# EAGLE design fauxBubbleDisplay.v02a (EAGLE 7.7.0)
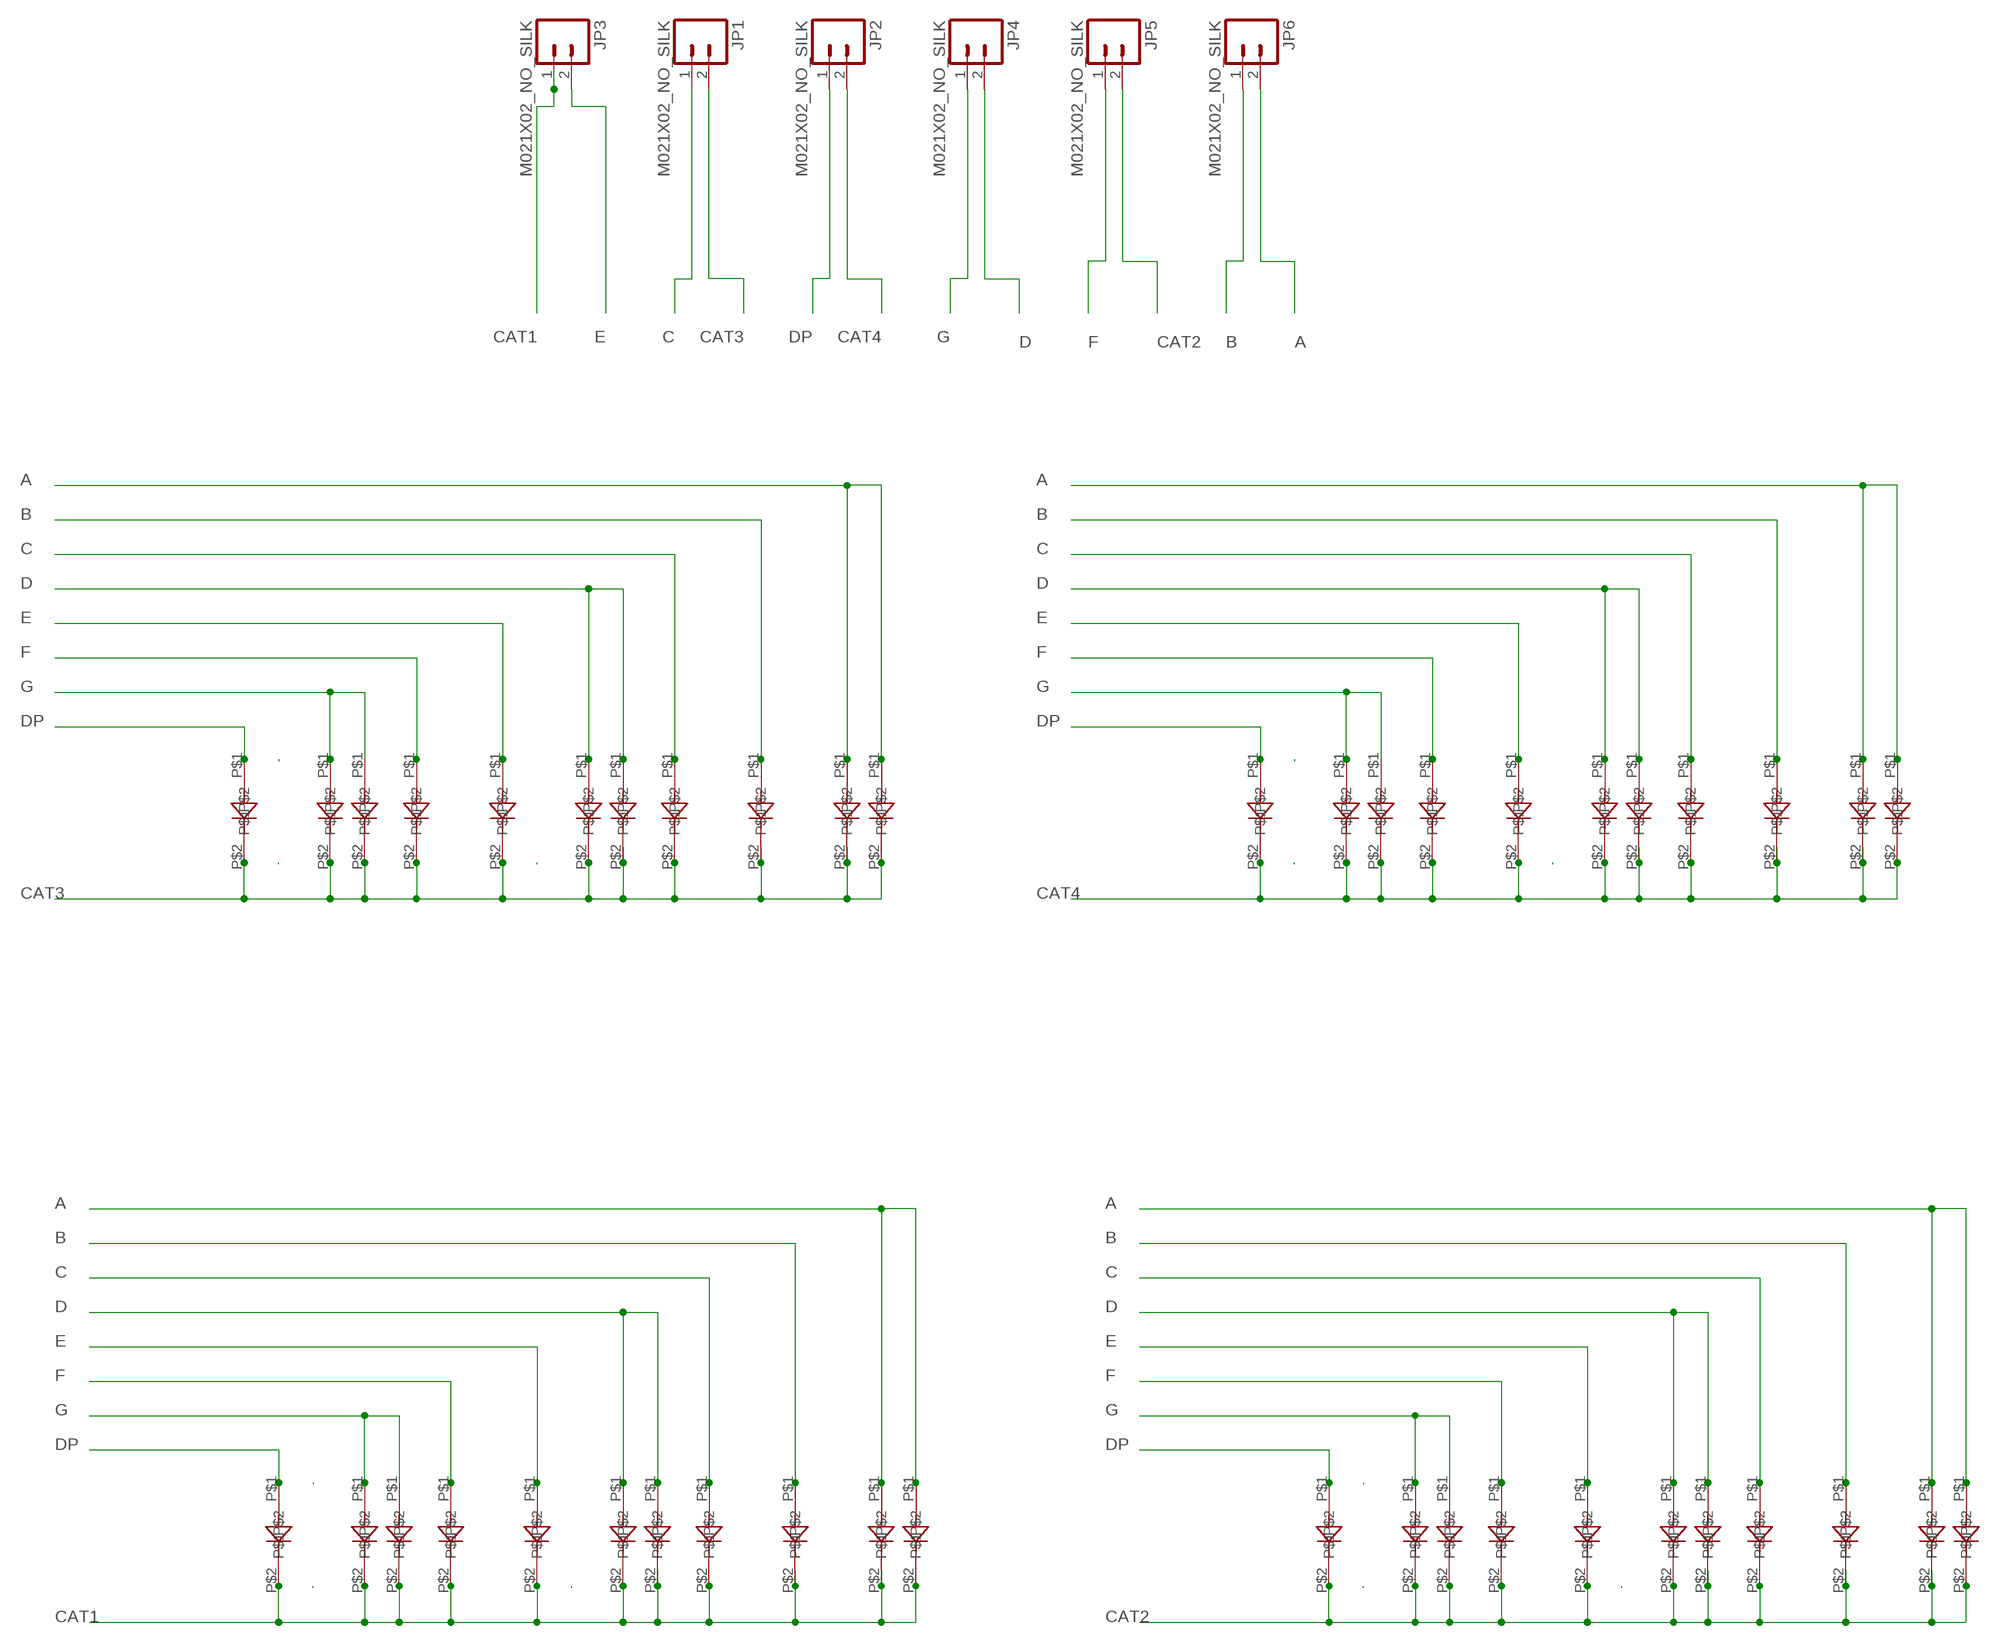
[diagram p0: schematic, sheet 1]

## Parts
JP1  M021X02_NO_SILK  [1X02_NO_SILK]
JP2  M021X02_NO_SILK  [1X02_NO_SILK]
JP3  M021X02_NO_SILK  [1X02_NO_SILK]
JP4  M021X02_NO_SILK  [1X02_NO_SILK]
JP5  M021X02_NO_SILK  [1X02_NO_SILK]
JP6  M021X02_NO_SILK  [1X02_NO_SILK]
U$1  LX201  [LX201]
U$2  LX201  [LX201]
U$3  LX201  [LX201]
U$4  LX201  [LX201]
U$5  LX201  [LX201]
U$6  LX201  [LX201]
U$7  LX201  [LX201]
U$8  LX201  [LX201]
U$9  LX201  [LX201]
U$10  LX201  [LX201]
U$11  LX201  [LX201]
U$12  LX201  [LX201]
U$13  LX201  [LX201]
U$14  LX201  [LX201]
U$15  LX201  [LX201]
U$16  LX201  [LX201]
U$17  LX201  [LX201]
U$18  LX201  [LX201]
U$19  LX201  [LX201]
U$20  LX201  [LX201]
U$21  LX201  [LX201]
U$22  LX201  [LX201]
U$23  LX201  [LX201]
U$24  LX201  [LX201]
U$25  LX201  [LX201]
U$26  LX201  [LX201]
U$27  LX201  [LX201]
U$28  LX201  [LX201]
U$29  LX201  [LX201]
U$30  LX201  [LX201]
U$31  LX201  [LX201]
U$32  LX201  [LX201]
U$33  LX201  [LX201]
U$34  LX201  [LX201]
U$35  LX201  [LX201]
U$36  LX201  [LX201]
U$37  LX201  [LX201]
U$38  LX201  [LX201]
U$39  LX201  [LX201]
U$40  LX201  [LX201]
U$41  LX201  [LX201]
U$42  LX201  [LX201]
U$43  LX201  [LX201]
U$44  LX201  [LX201]

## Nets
A: JP6.2 U$15.P$1 U$16.P$1 U$21.P$1 U$22.P$1 U$32.P$1 U$33.P$1 U$43.P$1 U$44.P$1
B: JP6.1 U$13.P$1 U$20.P$1 U$31.P$1 U$42.P$1
C: JP1.1 U$11.P$1 U$19.P$1 U$30.P$1 U$41.P$1
CAT1: JP3.1 U$1.P$2 U$2.P$2 U$4.P$2 U$5.P$2 U$7.P$2 U$9.P$2 U$10.P$2 U$11.P$2 U$13.P$2 U$15.P$2 U$16.P$2
CAT2: JP5.2 U$23.P$2 U$24.P$2 U$25.P$2 U$26.P$2 U$27.P$2 U$28.P$2 U$29.P$2 U$30.P$2 U$31.P$2 U$32.P$2 U$33.P$2
CAT3: JP1.2 U$3.P$2 U$6.P$2 U$8.P$2 U$12.P$2 U$14.P$2 U$17.P$2 U$18.P$2 U$19.P$2 U$20.P$2 U$21.P$2 U$22.P$2
CAT4: JP2.2 U$34.P$2 U$35.P$2 U$36.P$2 U$37.P$2 U$38.P$2 U$39.P$2 U$40.P$2 U$41.P$2 U$42.P$2 U$43.P$2 U$44.P$2
D: JP4.2 U$9.P$1 U$10.P$1 U$17.P$1 U$18.P$1 U$28.P$1 U$29.P$1 U$39.P$1 U$40.P$1
DP: JP2.1 U$4.P$1 U$8.P$1 U$25.P$1 U$36.P$1
E: JP3.2 U$7.P$1 U$14.P$1 U$27.P$1 U$38.P$1
F: JP5.1 U$5.P$1 U$12.P$1 U$26.P$1 U$37.P$1
G: JP4.1 U$1.P$1 U$2.P$1 U$3.P$1 U$6.P$1 U$23.P$1 U$24.P$1 U$34.P$1 U$35.P$1

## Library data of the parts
JP1-JP6 = SparkFun-Connectors:M02: Standard 2-pin 0.1" header. Use with
U$1-U$44 = kris:LX201

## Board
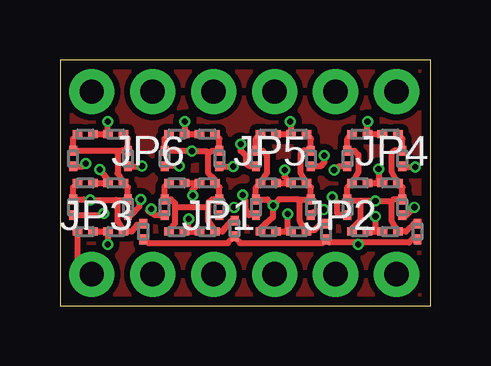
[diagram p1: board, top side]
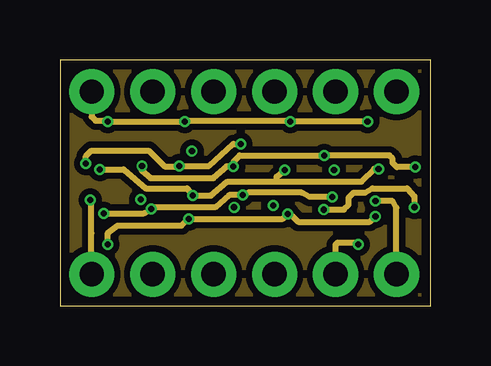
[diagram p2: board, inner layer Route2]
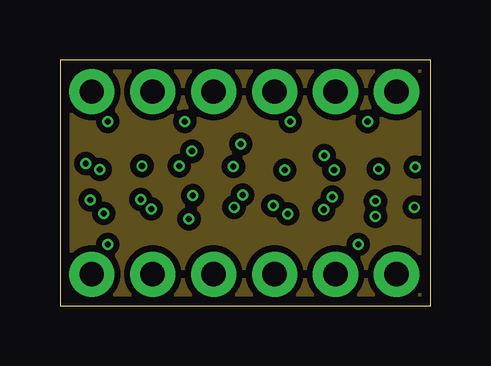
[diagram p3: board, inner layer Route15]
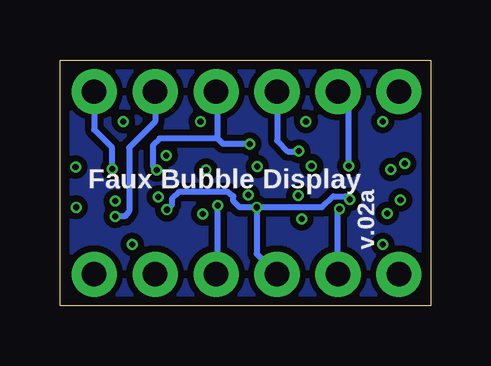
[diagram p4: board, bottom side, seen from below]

Size 15.44 x 10.26 mm. Coordinates in mm from the lower left corner, seen from the top.
Outline: 0,0 15.44,0 15.44,10.26 0,10.26 0,0
Copper layers (1*2*15*16): Top 0.035559375mm / dielectric 0.17018125mm / Route2 0.01778125mm / dielectric 47mil / Route15 0.01778125mm / dielectric 0.17018125mm / Bottom 0.035559375mm
Design rules "OSHPark-4layer *": minimum track width 5mil, minimum drill 10mil, track to track 5mil, track to pad 5mil, pad to pad 5mil, via to via 5mil, smd to smd 5mil, copper to edge 15mil, drill to drill 6mil, minimum pad ring 4mil, minimum via ring 4mil, stop-mask expansion 2.5mil, vias tented up to drill 20mil, thermal gap 10mil

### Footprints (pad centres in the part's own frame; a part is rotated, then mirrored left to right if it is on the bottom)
1X02_NO_SILK = drill 1.016 pad 1.88: 1 0,0; 2 2.54,0
LX201 = smd 0.4 x 0.33: P$1 -0.325,0; P$2 0.325,0

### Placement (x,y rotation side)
JP1  6.4,1.32 0 top
JP2  11.48,1.32 0 top
JP3  1.32,1.32 0 top
JP4  14.02,8.94 180 top
JP5  8.94,8.94 180 top
JP6  3.86,8.94 180 top
U$1  1.05,5.13 180 top
U$2  2.32,5.13 0 top
U$3  8.67,5.13 180 top
U$4  3.47,3.1 90 top
U$5  0.55,6.15 90 top
U$6  9.94,5.13 0 top
U$7  0.55,4.11 90 top
U$8  11.09,3.1 90 top
U$9  1.05,3.1 180 top
U$10  2.32,3.1 0 top
U$11  2.83,4.11 90 top
U$12  8.17,6.15 90 top
U$13  2.83,6.15 90 top
U$14  8.17,4.11 90 top
U$15  2.32,7.16 0 top
U$16  1.05,7.16 180 top
U$17  8.67,3.1 180 top
U$18  9.94,3.1 0 top
U$19  10.45,4.11 90 top
U$20  10.45,6.15 90 top
U$21  8.67,7.16 180 top
U$22  9.94,7.16 0 top
U$23  4.86,5.13 180 top
U$24  6.13,5.13 0 top
U$25  7.28,3.23 90 top
U$26  4.36,6.15 90 top
U$27  4.36,4.11 90 top
U$28  6.13,3.1 0 top
U$29  4.86,3.1 180 top
U$30  6.64,4.11 90 top
U$31  6.64,6.15 90 top
U$32  4.86,7.16 180 top
U$33  6.13,7.16 0 top
U$34  13.75,5.13 0 top
U$35  12.48,5.13 180 top
U$36  14.9,3.1 90 top
U$37  11.98,6.15 90 top
U$38  11.98,4.11 90 top
U$39  12.48,3.1 180 top
U$40  13.75,3.1 0 top
U$41  14.26,4.11 90 top
U$42  14.26,6.15 90 top
U$43  12.48,7.16 180 top
U$44  13.75,7.16 0 top

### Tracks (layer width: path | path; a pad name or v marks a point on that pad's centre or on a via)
A  (via drill 0.25)
  Top 0.254: v1.99,7.7 2,7.52 U$15.P$1 U$16.P$1 | v5.19,7.7 U$32.P$1 U$33.P$1 | U$21.P$1 U$22.P$1 9.61,7.67 v9.59,7.7 | U$44.P$1 U$43.P$1 12.81,7.61 v12.81,7.7
  Route2 0.254: v12.81,7.7 v9.59,7.7 9.51,7.72 5.35,7.72 5.22,7.77 v5.19,7.7 v1.99,7.7 1.97,7.72 1.49,7.72 1.32,7.89 JP6.2
B  (via drill 0.25)
  Top 0.254: U$13.P$1 3.4,5.82 v3.42,5.84 | U$31.P$1 v7.22,5.82 v7.23,5.82 | U$42.P$1 14.26,5.79 v14.8,5.79 | v11.01,6.27 11.01,5.99 10.86,5.82 U$20.P$1
  Route2 0.254: v14.8,5.79 14.03,5.79 13.86,5.97 13.86,6.15 13.73,6.27 v11.01,6.27 7.48,6.27 7.23,5.99 v7.23,5.82 6.95,5.82 6.39,5.33 3.77,5.33 3.42,5.64 v3.42,5.84
  Bottom 0.254: v3.42,5.84 3.42,8.5 JP6.1
C  (via drill 0.25)
  Top 0.254: U$41.P$1 14.45,3.79 v14.77,4.11 | v10.99,4.01 11.09,4.01 11.01,3.94 10.6,3.94 U$19.P$1 | U$30.P$1 6.75,3.79 7.1,4.11 v7.25,4.11 | U$11.P$1 2.96,3.79 3.32,4.17 3.32,4.37 v3.37,4.44
  Route2 0.254: v10.99,4.01 11.82,4.01 12.03,4.22 12.03,4.52 12.23,4.72 12.71,4.72 13.02,4.9 14.47,4.9 14.77,4.57 v14.77,4.11
  Bottom 0.254: v7.25,4.11 7.96,4.11 8.22,4.37 8.22,4.57 8.45,4.75 10.5,4.75 10.78,4.47 10.78,4.22 v10.99,4.01 | v3.37,4.44 3.54,4.57 4.05,4.57 4.53,4.11 v7.25,4.11 | v7.25,4.11 7.25,2.17 JP1.1
CAT1  (via drill 0.25)
  Top 0.254: U$1.P$2 0.55,4.95 U$7.P$2 1.01,4.44 v1.26,4.42 2.32,4.42 | U$4.P$2 3.47,3.38 3.21,3.38 2.98,3.1 U$10.P$2 2.4,3.53 2.4,4.34 2.32,4.42 | U$13.P$2 2.83,6.98 U$15.P$2 | U$16.P$2 0.55,6.98 U$5.P$2 U$13.P$2 | U$13.P$2 2.55,6.47 2.4,6.38 2.4,5.53 U$2.P$2 2.83,4.95 U$11.P$2 2.81,4.42 2.32,4.42 | U$9.P$2 0.73,1.91 JP3.1
  Route2 0.254: JP3.1 1.32,1.41 1.31,3.02 1.31,4.34 v1.26,4.42
CAT2  (via drill 0.25)
  Top 0.254: U$23.P$2 4.36,4.97 U$27.P$2 4.62,4.44 4.79,4.29 4.79,4.11 | U$33.P$2 6.64,6.98 U$31.P$2 6.34,6.48 6.19,6.38 | U$32.P$2 4.36,6.98 U$26.P$2 4.38,6.45 v5.5,6.45 6.11,6.45 6.19,6.38 | U$29.P$2 4.79,3.45 4.79,4.11 | U$25.P$2 7.15,3.55 6.77,3.1 U$28.P$2 6.21,3.47 6.19,3.58 6.19,4.11 | 6.19,6.38 6.19,5.54 6.46,5.26 U$24.P$2 6.64,4.95 U$30.P$2 6.36,4.44 6.19,4.32 6.19,4.11 | 6.19,4.11 4.79,4.11
  Bottom 0.254: JP5.2 6.4,6.89 5.96,6.45 5.52,6.45 v5.5,6.45
CAT3  (via drill 0.25)
  Top 0.254: U$21.P$2 8.17,6.98 U$12.P$2 8.45,6.47 8.62,6.3 8.62,5.56 U$3.P$2 8.17,4.95 U$14.P$2 8.64,4.44 v8.88,4.19 | U$22.P$2 10.45,6.98 U$20.P$2 10.14,6.47 10.02,6.35 10.02,5.56 U$6.P$2 10.45,4.95 U$19.P$2 9.94,4.44 | U$8.P$2 10.88,3.42 10.81,3.35 10.6,3.15 U$18.P$2 10.24,3.15 10,3.55 10,4.34 9.94,4.44 | 9.94,4.44 9.13,4.44 v8.88,4.19 | U$17.P$2 8.35,3.21 8.6,3.45 8.88,3.71 v8.88,4.19
  Bottom 0.254: v8.88,4.19 8.88,1.38 JP1.2
CAT4  (via drill 0.25)
  Top 0.254: U$43.P$2 11.98,6.98 U$37.P$2 12.26,6.47 12.43,6.3 12.43,5.58 U$35.P$2 11.98,4.95 U$38.P$2 12.1,4.37 12.56,4.37 | U$44.P$2 14.26,6.98 U$42.P$2 13.93,6.47 13.81,6.35 13.81,5.61 U$34.P$2 14.26,4.95 U$41.P$2 13.9,4.44 13.81,4.34 | 13.81,4.34 13.81,4.37 v13.14,4.37 12.56,4.37 | 13.81,4.34 13.81,3.55 U$40.P$2 14.41,3.1 14.74,3.42 U$36.P$2 | U$39.P$2 12.16,3.21 12.54,3.58 12.54,4.34 12.56,4.37
  Route2 0.254: JP2.2 14.02,4.09 13.86,4.37 v13.14,4.37
D  (via drill 0.25)
  Top 0.254: U$28.P$1 U$29.P$1 5.34,3.12 v5.37,3.63 | U$9.P$1 U$10.P$1 2,2.64 v1.99,2.57 | U$40.P$1 U$39.P$1 13.14,3.09 v13.14,3.73 | v9.49,3.84 9.49,3.23 U$18.P$1 U$17.P$1
  Route2 0.254: v1.99,2.57 1.99,3.05 2.4,3.35 5.07,3.35 v5.37,3.63 9.28,3.63 v9.49,3.84 9.59,3.84 9.92,3.5 12.92,3.5 v13.14,3.73
  Bottom 0.254: v13.14,3.73 13.11,3.74 12.73,3.73 12.56,3.96 12.56,6.6 11.48,7.68 JP4.2
DP  (via drill 0.25)
  Top 0.254: U$4.P$1 3.54,2.77 3.7,2.62 6.99,2.62 U$25.P$1 7.28,2.84 7.51,2.62 10.93,2.62 U$8.P$1 11.22,2.64 12.33,2.64 v12.43,2.57 12.51,2.64 14.54,2.64 14.67,2.77 U$36.P$1
  Route2 0.254: JP2.1 11.48,2.55 11.57,2.64 12.36,2.64 v12.43,2.57
E  (via drill 0.25)
  Top 0.254: v3.8,4.04 3.67,3.96 3.95,3.78 U$27.P$1 | U$7.P$1 1.75,3.79 v1.82,3.86 | U$14.P$1 7.88,3.79 7.73,4.04 7.73,4.39 v7.61,4.62 | U$38.P$1 11.67,3.79 11.54,3.89 11.54,4.32 v11.34,4.55
  Route2 0.254: v1.82,3.86 3.49,3.86 v3.8,4.04 3.9,4.11 6.46,4.11 7.05,4.62 v7.61,4.62 7.84,4.72 10.07,4.72 10.4,4.55 v11.34,4.55
  Bottom 0.254: JP3.2 3.86,3.97 v3.8,4.04
F  (via drill 0.25)
  Top 0.254: U$5.P$1 0.96,5.82 v1.08,5.94 | v4.97,5.84 4.46,5.84 U$26.P$1 | v7.53,6.76 7.53,6.48 7.73,6.27 7.73,5.94 7.89,5.84 8.12,5.84 U$12.P$1 | U$37.P$1 11.63,5.82 v11.42,5.66
  Route2 0.254: v1.08,5.94 1.08,6.25 1.31,6.48 3.7,6.48 3.9,6.27 4,6.18 U$26.P$1 4.88,5.82 v4.97,5.84 6.21,5.84 7.23,6.76 v7.53,6.76
  Bottom 0.254: v7.53,6.76 8.65,6.76 8.88,6.98 | 8.88,6.98 8.88,8.88 JP5.1 | 8.88,6.98 11.29,6.98 11.57,6.71 11.57,5.82 v11.42,5.66
G  (via drill 0.25)
  Top 0.254: U$23.P$1 U$24.P$1 5.52,4.85 v5.52,4.6 | U$1.P$1 U$2.P$1 2,5.28 v1.66,5.69 | U$3.P$1 U$6.P$1 9.36,5.39 v9.36,5.66 | U$35.P$1 U$34.P$1 13.27,5.29 v13.27,5.71
  Route2 0.254: 9.03,5.18 6.97,5.18 6.29,4.6 v5.52,4.6 5.3,4.9 3.57,4.9 2.65,5.69 v1.66,5.69 | 9.03,5.18 12.56,5.18 13.09,5.71 v13.27,5.71 | 9.03,5.18 9.03,5.38 v9.36,5.66
  Bottom 0.254: v13.27,5.71 13.27,6.6 14.02,7.35 JP4.1
GND
  pour Top (isolate 0.254, no thermals): -0.01,10.26 15.48,10.26 15.48,0 -0.01,0
  pour Bottom (isolate 0.254, no thermals): -0.01,10.26 15.51,10.26 15.51,0 -0.01,0
  pour Route15 (isolate 0.254, no thermals): -0.04,10.26 15.48,10.26 15.48,0 -0.01,0 -0.01,8.31
  pour Route2 (isolate 0.254, no thermals): -0.06,10.26 15.46,10.26 15.46,0 -0.01,0 -0.01,8.31

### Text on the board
bPlace: v.02a | Faux Bubble Display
